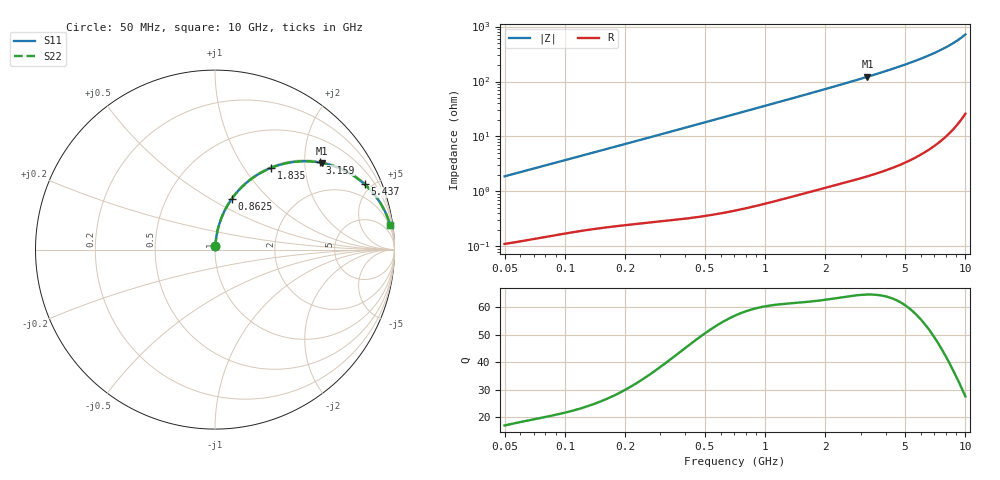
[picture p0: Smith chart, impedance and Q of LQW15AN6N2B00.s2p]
!Murata Part Number: LQW15AN6N2B00
!These Parameters are Measured in Series Mode Connection
!  o--[Z]--o
!Port1  Port2
!  o-------o
!Freq. Start=50[MHz] Stop=10[GHz], 401[Steps]
# Hz S RI R 50
!Freq.(Hz)	S 11(Real)	S 11(Imag)	S 21(Real)	S 21(Imag)	S 12(Real)	S 12(Imag)	S 22(Real)	S 22(Imag)
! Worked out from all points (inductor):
!   401 points, 50 MHz to 10 GHz, reference 50 ohm
!   read as one part in series: L = 5.96 nH near 51.34 MHz
!   highest Q = 64.6 at 3.244 GHz (marker M1), where L = 5.98 nH
!   S11 on the Smith chart (normalised r, x): 50 MHz: 1.00, +0.04; 862.5 MHz: 1.01, +0.62; 1.835 GHz: 1.02, +1.34; 3.159 GHz: 1.04, +2.37; 5.437 GHz: 1.08, +4.54; 10 GHz: 2, +14
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5e7  0.00146 0.0188  0.9985 -0.0188  0.9985 -0.0188  0.00146 0.0188
1.214486e8  0.00391 0.0445  0.9961 -0.0445  0.9961 -0.0445  0.00391 0.0445
1.956524e8  0.00745 0.0707  0.9925 -0.0707  0.9925 -0.0707  0.00745 0.0707
2.949953e8  0.0141 0.1053  0.9859 -0.1053  0.9859 -0.1053  0.0141 0.1053
4.628099e8  0.0304 0.1618  0.9696 -0.1618  0.9696 -0.1618  0.0304 0.1618
7.071068e8  0.065 0.2378  0.935 -0.2378  0.935 -0.2378  0.065 0.2378
8.625288e8  0.0925 0.2814  0.9075 -0.2814  0.9075 -0.2814  0.0925 0.2814
1.038268e9  0.1275 0.3254  0.8725 -0.3254  0.8725 -0.3254  0.1275 0.3254
1.233369e9  0.1701 0.3676  0.8299 -0.3676  0.8299 -0.3676  0.1701 0.3676
1.465132e9  0.2237 0.4087  0.7763 -0.4087  0.7763 -0.4087  0.2237 0.4087
1.717543e9  0.2835 0.4427  0.7165 -0.4427  0.7165 -0.4427  0.2835 0.4427
1.835145e9  0.3113 0.4551  0.6887 -0.4551  0.6887 -0.4551  0.3113 0.4551
2.423676e9  0.4436 0.489  0.5564 -0.489  0.5564 -0.489  0.4436 0.489
2.766943e9  0.5126 0.4921  0.4874 -0.4921  0.4874 -0.4921  0.5126 0.4921
3.158828e9  0.5827 0.4854  0.4173 -0.4854  0.4173 -0.4854  0.5827 0.4854
3.243629e9  0.5966 0.4829  0.4034 -0.4829  0.4034 -0.4829  0.5966 0.4829
4.171863e9  0.7225 0.44  0.2775 -0.44  0.2775 -0.44  0.7225 0.44
5.437278e9  0.8333 0.3643  0.1667 -0.3643  0.1667 -0.3643  0.8333 0.3643
6.54512e9  0.8933 0.2993  0.1067 -0.2993  0.1067 -0.2993  0.8933 0.2993
7.672705e9  0.9329 0.2392  0.0671 -0.2392  0.0671 -0.2392  0.9329 0.2392
8.644138e9  0.9557 0.1928  0.0443 -0.1928  0.0443 -0.1928  0.9557 0.1928
1e10  0.9762 0.1354  0.0238 -0.1354  0.0238 -0.1354  0.9762 0.1354
